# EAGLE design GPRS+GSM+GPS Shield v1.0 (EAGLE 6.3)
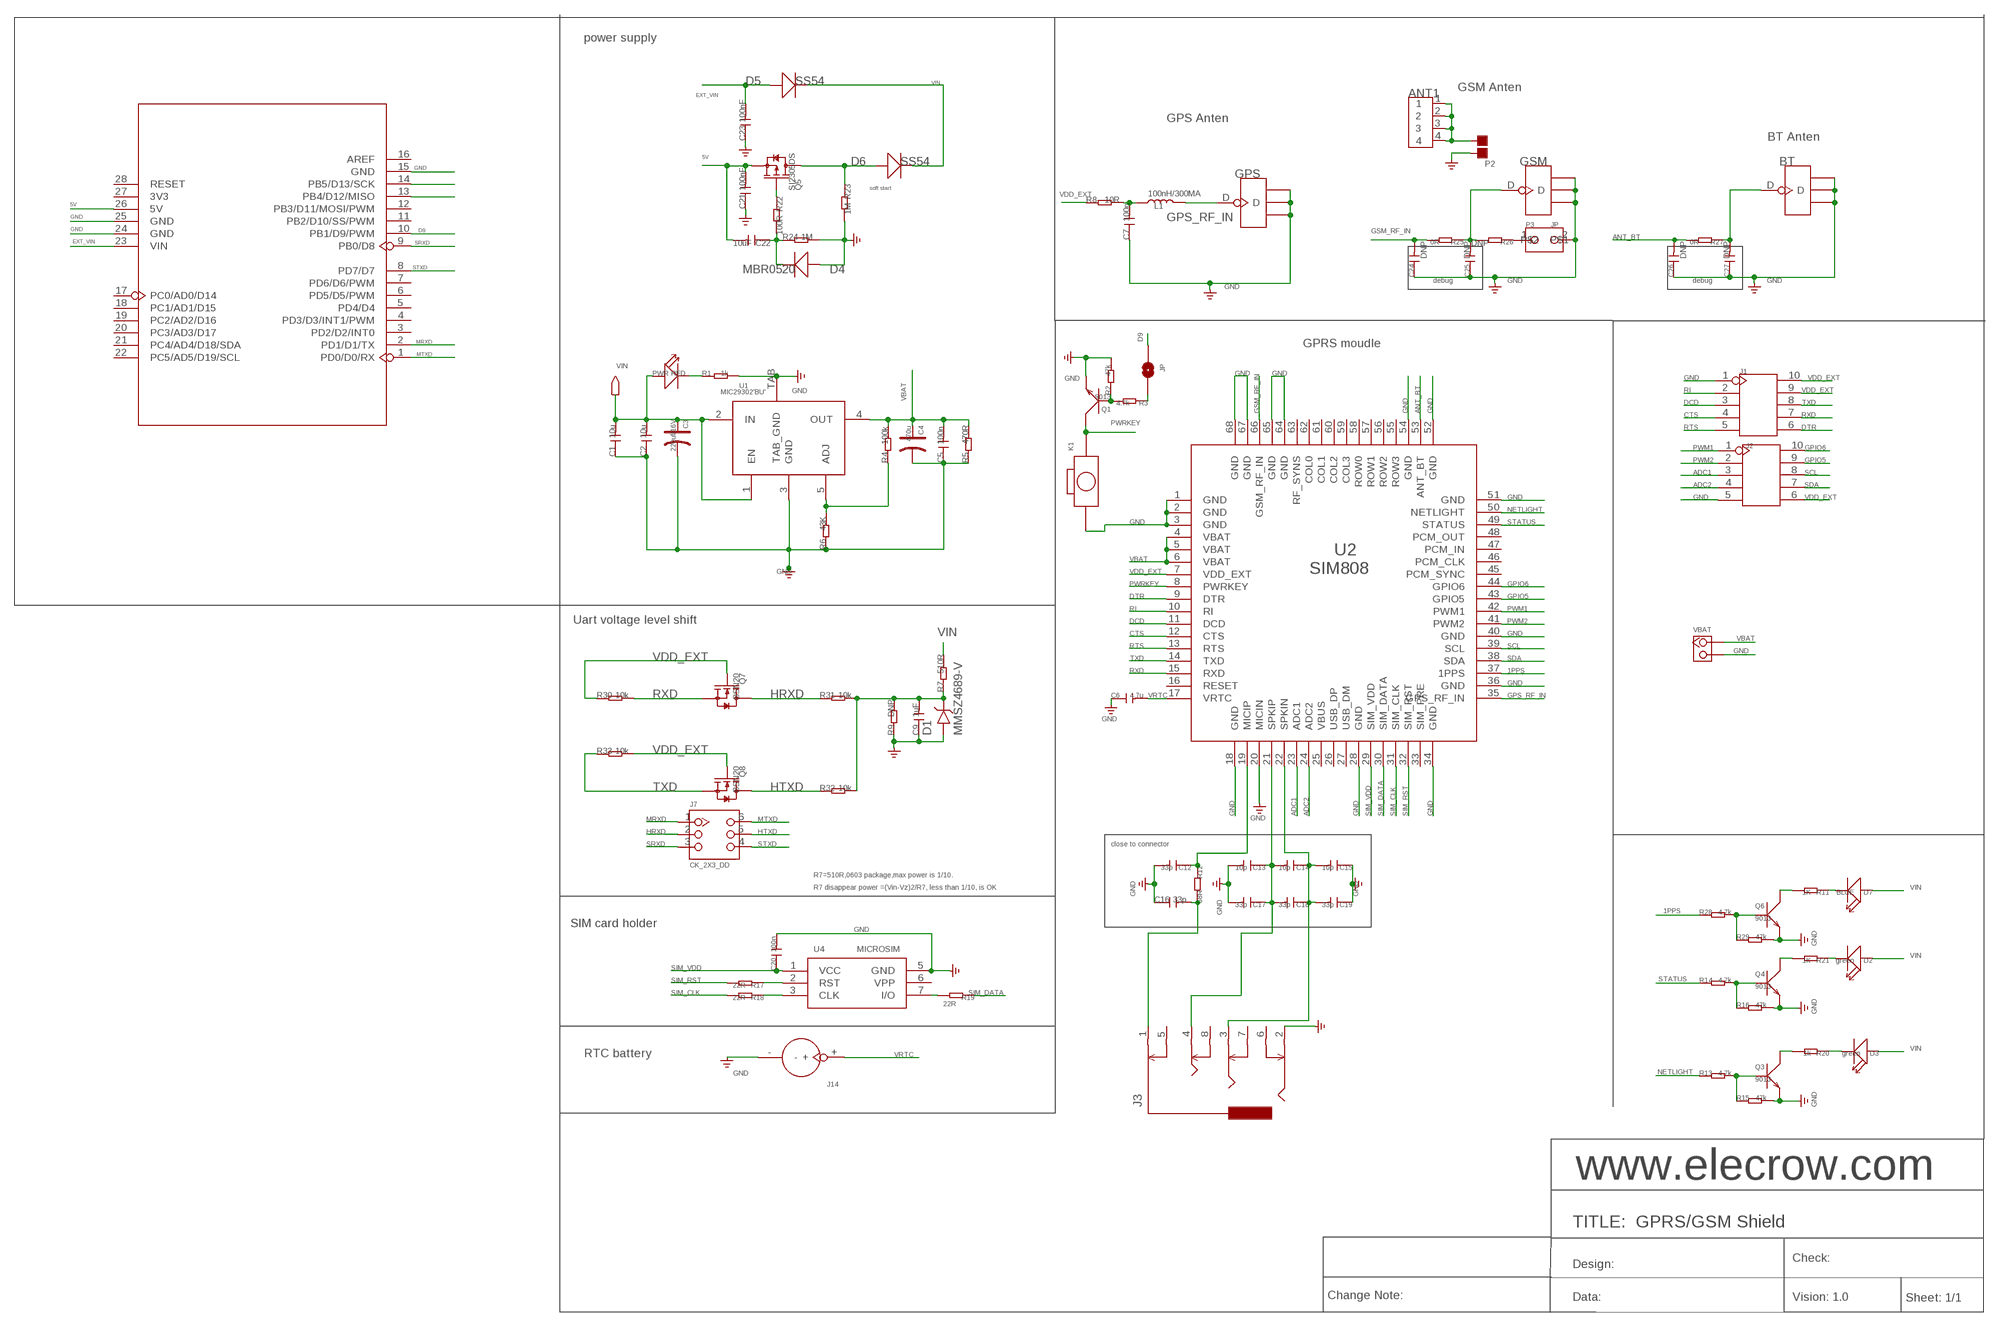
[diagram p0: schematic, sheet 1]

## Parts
ANT1  ANTENNA-SMA-IPX  [SMA-TO-IPX]
BT  ANTENNA-U-FL  [4P-U-FL]
C1  10u  C-0603  [C0603]
C2  10u  C-0603  [C0603]
C3  220uf/16V  006-CAP_AVX_D  [AVX_D]
C4  470u  006-CAP_AVX_D  [AVX_D]
C5  100n  C-0603  [C0603]
C6  4.7u  C-0805  [C0805]
C7  100n  C-0603  [C0603]
C9  1uF  C-0603  [C0603]
C12  33p  C-0603  [C0603]
C13  10p  C-0402  [C0402]
C14  10p  C-0402  [C0402]
C15  10p  C-0402  [C0402]
C16  33p  C-0603  [C0603]
C17  33p  C-0402  [C0402]
C18  33p  C-0402  [C0402]
C19  33p  C-0402  [C0402]
C20  100n  C-0603  [C0603]
C21  100nF  C-0603  [C0603]
C22  10uF  C-0805  [C0805]
C23  100nF  C-0603  [C0603]
C24  DNP  C-0402  [C0402]
C25  DNP  C-0402  [C0402]
C26  DNP  C-0402  [C0402]
C27  DNP  C-0402  [C0402]
D1  MMSZ4689-V  D-VOL'MMSZ4681'  [SOD123-2.7X1.6]
D2  green  LED'0603'  [LED-0603]
D3  green  LED'0603'  [LED-0603]
D4  MBR0520  D'MBR0520LT1'  [SOD123-2.7X1.6]
D5  SS54  D'MBRS240LT3'  [SMB]
D6  SS54  D'MBRS240LT3'  [SMB]
D7  BLUE  LED'0603'  [LED-0603]
GPS  ANTENNA-U-FL  [4P-U-FL]
GSM  ANTENNA-U-FL  [4P-U-FL]
J1  HEADER-2X5P-2.54  [2X5P-2.54]
J2  HEADER-2X5P-2.54  [2X5P-2.54]
J3  AUDIO-8P'PJ-3536-L6S'  [8P-3.5-SMD]
J7  CK_2X3_DD  [CK_2X3]
J14  HOLDER-BATTERY-2P-CR1220  [CR1220]
JP  0R/0805  PAD-SOLDERJUMPERNC  [2P-SMD-3.3X2]
K1  BOTTON_1_DP  [BTN_5.0_RST]
L1  100nH/300MA  L'0603'  [L0603]
P2  PAD-JUMPER-2P  [2P-SMD-1.78X1.27]
P3  JP  [JP]
PWR  RED  007-LED0603  [D0603]
Q1  9013  TRANSISTOR-NPN-SOT23  [SOT23]
Q3  9013  TRANSISTOR-NPN-SOT23  [SOT23]
Q4  9013  TRANSISTOR-NPN-SOT23  [SOT23]
Q5  SI2305DS  MOSFET-P'SI2323CDS/SI2305DS<BR>'  [SOT23]
Q6  9013  TRANSISTOR-NPN-SOT23  [SOT23]
Q7  BSN20  MOSFET-N'SOT23'  [SOT23]
Q8  BSN20  MOSFET-N'SOT23'  [SOT23]
R1  1k  R-0603  [R0603]
R2  47k  R-0603  [R0603]
R3  4.7k  R-0603  [R0603]
R4  100k  R-0603  [R0603]
R5  470R  R-0603  [R0603]
R6  43K  R-0603  [R0603]
R7  510R  R-0603  [R0603]
R8  10R  R-0603  [R0603]
R9  DNP  R-0603  [R0603]
R11  1K  R-0603  [R0603]
R12  68R  R-0603  [R0603]
R13  4.7k  R-0603  [R0603]
R14  4.7k  R-0603  [R0603]
R15  47k  R-0603  [R0603]
R16  47k  R-0603  [R0603]
R17  22R  R-0603  [R0603]
R18  22R  R-0603  [R0603]
R19  22R  R-0603  [R0603]
R20  1k  R-0603  [R0603]
R21  1K  R-0603  [R0603]
R22  100R  R-0603  [R0603]
R23  1M  R-0603  [R0603]
R24  1M  R-0603  [R0603]
R25  0R  R-0402  [R0402]
R26  DNP  R-0402  [R0402]
R27  0R  R-0402  [R0402]
R28  4.7k  R-0603  [R0603]
R29  47k  R-0603  [R0603]
R30  10k  R-0603  [R0603]
R31  10k  R-0603  [R0603]
R32  10k  R-0603  [R0603]
R33  10k  R-0603  [R0603]
U1  MIC29302'BU'  [TO-263]
U2  SIM808  [SIM808]
U3  UNO-SHILED  [SHILED]
U4  MICROSIM  [MICROSIM]
VBAT  DNP  HEADER_1X2_2.54  [CK_1*2]

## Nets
1PPS: R28.1 U2.37(1PPS)
5V: C21.2 C22.2 Q5.2(S) U3.26(5V)
ADC1: J2.3 U2.23(ADC1)
ADC2: J2.4 U2.24(ADC2)
ANT_BT: C26.2 R27.2 U2.53(ANT_BT)
CTS: J1.4 U2.12(CTS)
D9: JP.1 U3.10(PB1/D9/PWM)
DCD: J1.3 U2.11(DCD)
DTR: J1.6 U2.9(DTR)
EXT_VIN: C23.2 D5.+ U3.23(VIN)
GND: BT.GND1 BT.GND2 BT.GND3 C1.1 C2.1 C3.- C4.- C5.1 C6.1 C7.1 C9.1 C12.2 C13.2 C15.1 C16.1 C17.2 C19.1 C20.2 C21.1 C23.1 C24.1 C25.1 C26.1 C27.1 D1.1 D4.1(+) GPS.GND1 GPS.GND2 GPS.GND3 GSM.GND1 GSM.GND2 GSM.GND3 J1.1 J2.5 J3.2 J14.- K1.P$1 P2.2 P3.2 Q1.2(E) Q3.2(E) Q4.2(E) Q6.2(E) R1.2 R2.2 R5.1 R6.1 R9.1 R15.2 R16.2 R23.2 R24.2 R29.2 U1.3(GND) U1.TAB(TAB_GND) U2.1(GND) U2.2(GND) U2.3(GND) U2.18(GND) U2.20(MICIN) U2.28(GND) U2.34(GND) U2.36(GND) U2.40(GND) U2.51(GND) U2.52(GND) U2.54(GND) U2.64(GND) U2.65(GND) U2.67(GND) U2.68(GND) U3.15(GND) U3.24(GND) U3.25(GND) U4.5(GND) VBAT.2
GPIO5: J2.9 U2.43(GPIO5)
GPIO6: J2.10 U2.44(GPIO6)
GPS_RF_IN: GPS.D L1.2 U2.35(GPS_RF_IN)
GSM_RF_IN: C24.2 R25.2 U2.66(GSM_RF_IN)
HRXD: J7.2 Q7.3(D) R31.1
HTXD: J7.5 Q8.3(D) R32.1
MRXD: J7.1 U3.2(PD1/D1/TX)
MTXD: J7.6 U3.1(PD0/D0/RX)
N$1: R19.2 U4.7(I/O)
N$2: R4.1 R6.2 U1.5(ADJ)
N$3: Q3.3(C) R20.2
N$4: Q6.3(C) R11.2
N$5: R18.1 U4.3(CLK)
N$6: R17.1 U4.2(RST)
N$7: D3.- R20.1
N$8: Q3.1(B) R13.2 R15.1
N$9: C9.2 D1.2 R7.1 R9.2 R31.2 R32.2
N$11: Q5.1(G) R22.1
N$12: ANT1.1 ANT1.2 ANT1.3 ANT1.4 P2.1
N$13: C12.1 R12.1 U2.19(MICIP)
N$14: JP.2 R3.1
N$15: C13.1 C14.2 C17.1 C18.2 J3.4 U2.21(SPKIP)
N$16: Q4.3(C) R21.2
N$17: D2.- R21.1
N$18: Q4.1(B) R14.2 R16.1
N$19: C14.1 C15.2 C18.1 C19.2 J3.3 U2.22(SPKIN)
N$20: D6.+ Q5.3(D) R23.1
N$21: C7.2 L1.1 R8.2
N$22: D7.- R11.1
N$23: U3.14(PB5/D13/SCK)
N$24: Q6.1(B) R28.2 R29.1
N$25: C25.2 GSM.D R25.1 R26.2
N$26: P3.1 R26.1
N$27: U3.13(PB4/D12/MISO)
N$28: BT.D C27.2 R27.1
N$30: C16.2 J3.1 R12.2
N$36: Q1.1(B) R2.1 R3.2
N$39: C22.1 D4.2(-) R22.2 R24.1
N$53: PWR.- R1.1
NETLIGHT: R13.1 U2.50(NETLIGHT)
PWM1: J2.1 U2.42(PWM1)
PWM2: J2.2 U2.41(PWM2)
PWRKEY: K1.P$2 Q1.3(C) U2.8(PWRKEY)
RI: J1.2 U2.10(RI)
RTS: J1.5 U2.13(RTS)
RXD: J1.7 Q7.2(S) R30.2 U2.15(RXD)
SCL: J2.8 U2.39(SCL)
SDA: J2.7 U2.38(SDA)
SIM_CLK: R18.2 U2.31(SIM_CLK)
SIM_DATA: R19.1 U2.30(SIM_DATA)
SIM_RST: R17.2 U2.32(SIM_RST)
SIM_VDD: C20.1 U2.29(SIM_VDD) U4.1(VCC)
SRXD: J7.3 U3.9(PB0/D8)
STATUS: R14.1 U2.49(STATUS)
STXD: J7.4 U3.8(PD7/D7)
TXD: J1.8 Q8.2(S) R33.1 U2.14(TXD)
VBAT: C4.+ C5.2 R4.2 R5.2 U1.4(OUT) U2.4(VBAT) U2.5(VBAT) U2.6(VBAT) VBAT.1
VDD_EXT: J1.9 J1.10 J2.6 Q7.1(G) Q8.1(G) R8.1 R30.1 R33.2 U2.7(VDD_EXT)
VIN: C1.2 C2.2 C3.+ D2.+ D3.+ D5.- D6.- D7.+ PWR.+ R7.2 U1.1(EN) U1.2(IN)
VRTC: C6.2 J14.+ U2.17(VRTC)
Unconnected: J3.5 J3.6 J3.7 J3.8 U2.16(RESET) U2.25(VBUS) U2.26(USB_DP) U2.27(USB_DM) U2.33(SIM_PRE) U2.45(PCM_SYNC) U2.46(PCM_CLK) U2.47(PCM_IN) U2.48(PCM_OUT) U3.3(PD2/D2/INT0) U3.4(PD3/D3/INT1/PWM) U3.5(PD4/D4) U3.6(PD5/D5/PWM) U3.7(PD6/D6/PWM) U3.11(PB2/D10/SS/PWM) U3.12(PB3/D11/MOSI/PWM) U3.16(AREF) U3.17(PC0/AD0/D14) U3.18(PC1/AD1/D15) U3.19(PC2/AD2/D16) U3.20(PC3/AD3/D17) U3.21(PC4/AD4/D18/SDA) U3.22(PC5/AD5/D19/SCL) U3.27(3V3) U3.28(RESET) U4.6(VPP)

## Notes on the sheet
- power supply
- GSM Anten
- GPS Anten
- BT Anten
- soft start
- debug | debug
- GPRS moudle
- Uart voltage level shift
- close to connector
- R7=510R,0603 package,max power is 1/10.
- R7 disappear power =(Vin-Vz)2/R7, less than 1/10, is OK
- SIM card holder
- RTC battery
- www.elecrow.com
- TITLE:  GPRS/GSM Shield
- Check:
- Design:
- Change Note: | Data: | Vision: 1.0 | Sheet: 1/1

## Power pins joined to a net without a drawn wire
COL0: U2.62(COL0)
COL1: U2.61(COL1)
COL2: U2.60(COL2)
COL3: U2.59(COL3)
RF_SYNS: U2.63(RF_SYNS)
ROW0: U2.58(ROW0)
ROW1: U2.57(ROW1)
ROW2: U2.56(ROW2)
ROW3: U2.55(ROW3)

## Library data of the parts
ANT1 = Connector:ANTENNA-SMA-IPX
BT GPS GSM = Connector:ANTENNA-U-FL
C1 C2 C5-C7 C9 C12-C27 = Discrete:C*: Ceramic Capacitors
C3 C4 = Discrete:006-CAP*: Electrolytic Capacitors,Tantalum Capacitors and Super Capacitors
D1 = template:D-VOL
D2 D3 D7 = Discrete:LED*
D4-D6 = Discrete:D*
J1 J2 = Connector:HEADER-2X5P
J3 = template:AUDIO-8P
J7 = CONNECTER:CK_2X3
J14 = Connector:HOLDER-BATTERY-2P
JP = Discrete:PAD-SOLDERJUMPER: Solder Jumper
K1 = CPT_SMD:BOTTON_1
L1 = Discrete:L*
P2 = Discrete:PAD-JUMPER-2P; PARTNO: DNP
P3 = mySeeed:JP
PWR = Discrete:007-LED*
Q1 Q3 Q4 Q6 = Discrete:TRANSISTOR-NPN*: NPN audion
Q5 = Discrete:MOSFET-P
Q7 Q8 = Discrete:MOSFET-N: IRLL014: http://www.vishay.com/docs/91319/sihll014.pdf
R1-R9 R11-R33 = Discrete:R*
U1 = ICs_v54:MIC29302
U2 = moudle:SIM808
U3 = ljb:UNO-SHILED
U4 = Connector:MICROSIM
VBAT = CONNECTER:HEADER_1X2

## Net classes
0 default: width 0.152 mm, drill 0.152 mm, clearance 0.152 mm

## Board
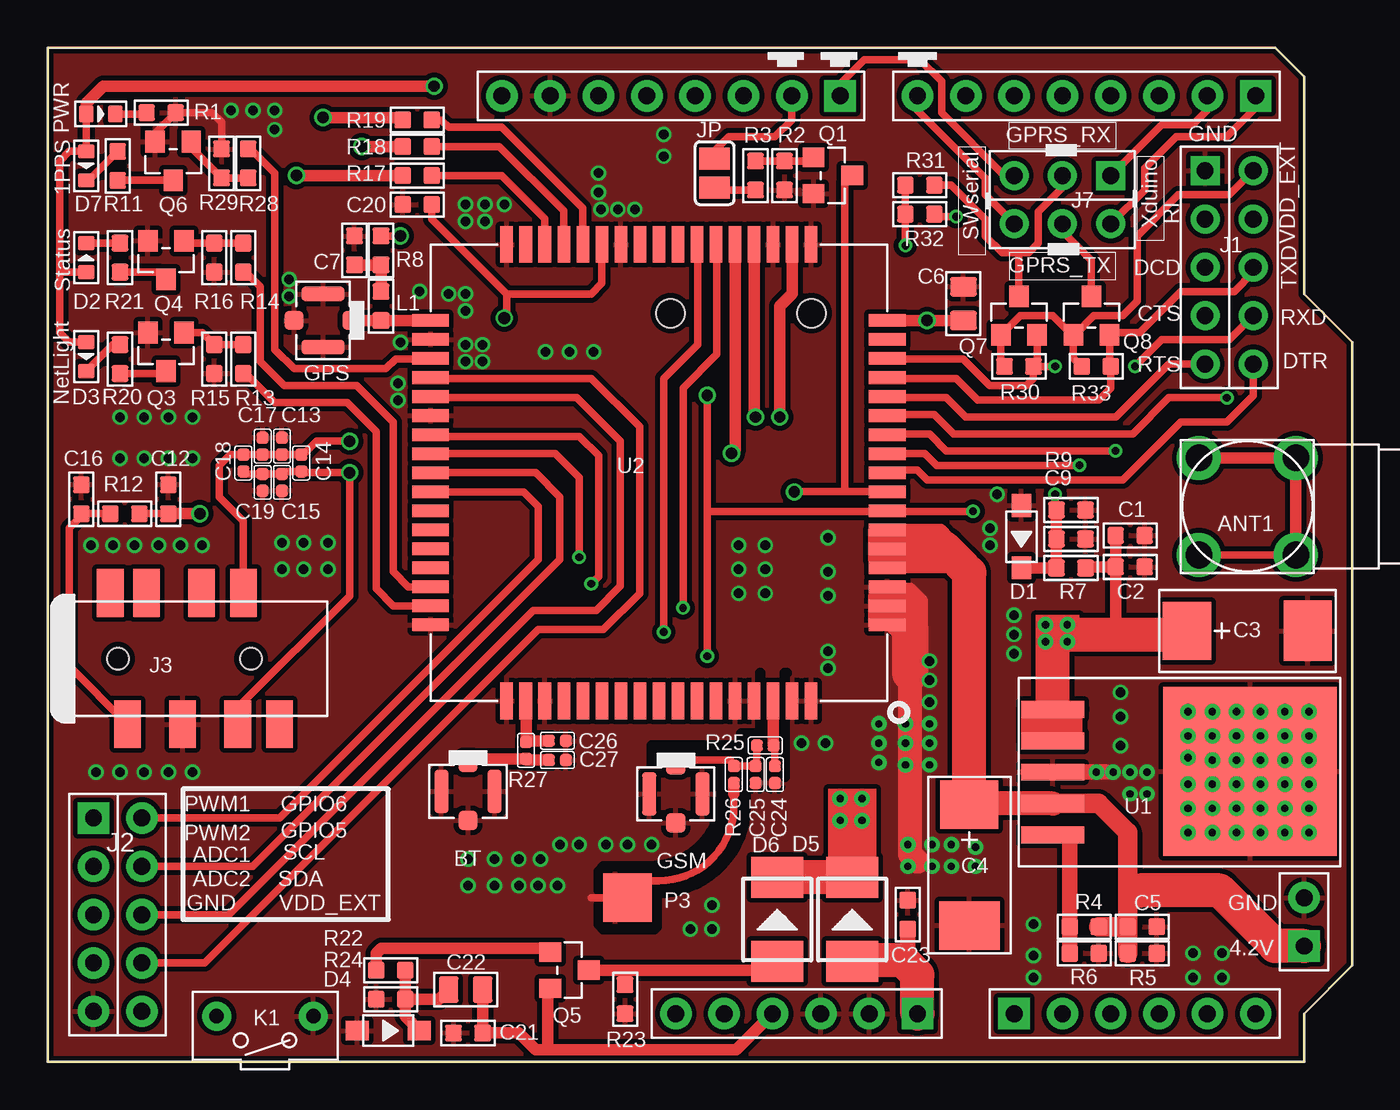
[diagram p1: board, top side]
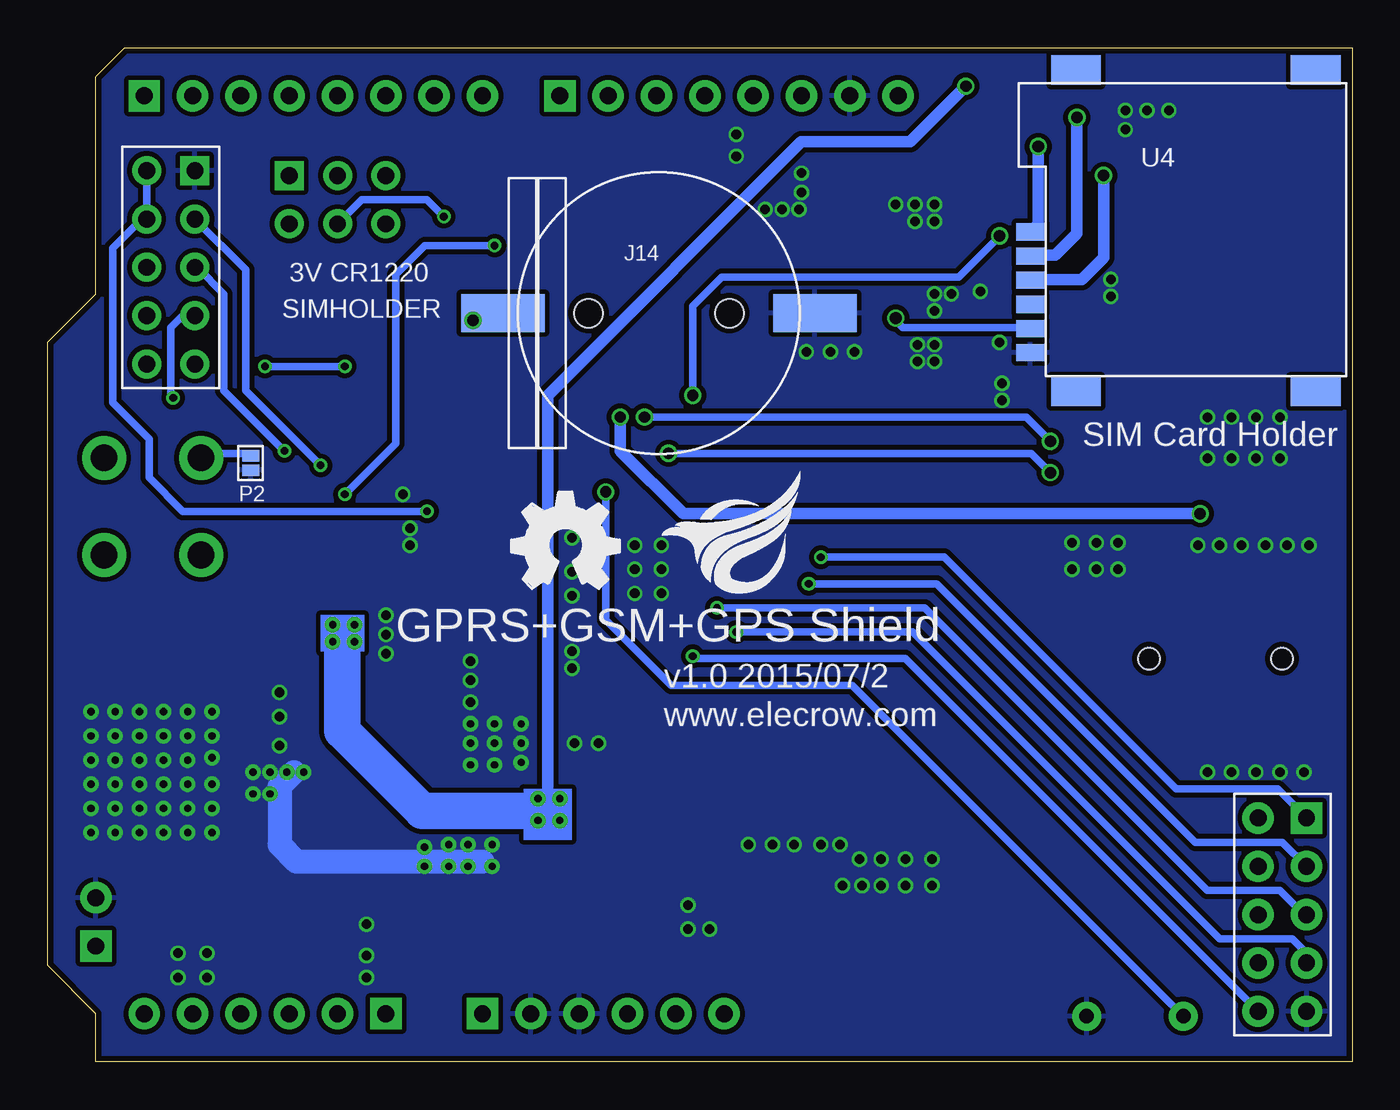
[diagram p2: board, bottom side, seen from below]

Size 68.58 x 53.34 mm. Coordinates in mm from the lower left corner, seen from the top.
Outline: 0,0 66.04,0 66.04,2.54 68.58,5.08 68.58,37.85 66.04,40.39 66.04,51.82 64.52,53.34 0,53.34 0,0
Copper layers (1*16): Top 0.035mm / dielectric 1.5mm / Bottom 0.035mm
Design rules "default *": minimum track width 6mil, minimum drill 12mil, track to track 10mil, track to pad 10mil, pad to pad 10mil, via to via 6mil, smd to smd 0mil, copper to edge 12mil, drill to drill 12mil, minimum pad ring 10mil, minimum via ring 6mil, stop-mask expansion 2mil, vias tented up to drill 100mil, thermal gap 10mil
tRestrict: area 35.6,41.9 to 35.7,43.3; 19 lines

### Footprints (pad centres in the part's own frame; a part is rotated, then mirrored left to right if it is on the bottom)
SMA-TO-IPX = drill 1.4 pad 2.3: 1 -2.55,2.55; 2 2.55,2.55; 3 2.55,-2.55; 4 -2.55,-2.55
4P-U-FL = smd 1.016 x 1.016: D -1.524,0; GND3 1.524,0 | smd 2.286 x 0.762: GND1 0,1.397; GND2 0,-1.397
C0603 = smd 0.889 x 0.889: 1 -0.762,0; 2 0.762,0
AVX_D = smd 2.54 x 3.048: + -3.175,0 | smd 2.54 x 3.175: - 3.175,0
C0805 = smd 1.016 x 1.397: 1 -0.889,0; 2 0.889,0
C0402 = smd 0.635 x 0.635: 1 -0.445,0; 2 0.445,0
SOD123-2.7X1.6 = smd 1.2 x 1.02: 1 -1.635,0; 2 1.635,0
D0603 = smd 0.762 x 0.889: + -0.762,0; - 0.762,0
SMB = smd 2.159 x 2.743: + -2.21,0; - 2.21,0
LED-0603 = smd 0.762 x 0.889: + -0.762,0; - 0.762,0
U-FL = smd 1.016 x 1.016: D -1.524,0; GND3 1.524,0 | smd 2.286 x 0.762: GND1 0,1.397; GND2 0,-1.397
2X5P-2.54-LEADED = drill 0.889 pad 1.524 square: 1 -1.27,5.08 | drill 0.889 pad 1.524: 2 -1.27,2.54; 3 -1.27,0; 4 -1.27,-2.54; 5 -1.27,-5.08; 6 1.27,-5.08; 7 1.27,-2.54; 8 1.27,0; 9 1.27,2.54; 10 1.27,5.08
2X5P-2.54 = drill 0.889 pad 1.651 square: 1 -1.27,5.08 | drill 0.889 pad 1.651: 2 -1.27,2.54; 3 -1.27,0; 4 -1.27,-2.54; 5 -1.27,-5.08; 6 1.27,-5.08; 7 1.27,-2.54; 8 1.27,0; 9 1.27,2.54; 10 1.27,5.08
8P-3.5-SMD = smd 1.4 x 2.5: 1 2.8,-3.45; 2 5.7,-3.45; 3 8.6,-3.45; 4 8.9,3.45; 5 1.9,3.45; 6 3.8,3.45; 7 6.7,3.45; 8 10.8,-3.45 | hole 1.149: 2.3,0; 9.3,0
CK_2X3 = drill 0.889 pad 1.524 square: 1 -1.27,2.54 | drill 0.889 pad 1.524: 2 -1.27,0; 3 -1.27,-2.54; 4 1.27,-2.54; 5 1.27,0; 6 1.27,2.54
CR1220 = smd 2 x 4.4: + 0,-8.2; - 0,8.2 | hole 1.5: 0,3.7; 0,-3.7
2P-SMD-3.3X2 = smd 1.168 x 1.6: 1 -0.762,0; 2 0.762,0
BTN_5.0_RST = drill 0.762 pad 1.524: P$1 0,2.54; P$2 0,-2.54
L0603 = smd 0.889 x 0.889: 1 -0.762,0; 2 0.762,0
2P-SMD-1.78X1.27 = smd 0.889 x 0.61: 1 0,0.381; 2 0,-0.381
JP = smd 1.27 x 2.54: 1 -0.635,0; 2 0.635,0
SOT23 = smd 1.016 x 1.143: 1 -0.95,-1.016; 2 0.95,-1.016; 3 0,1.016
R0603 = smd 0.889 x 0.889: 1 -0.762,0; 2 0.762,0
R0402 = smd 0.635 x 0.635: 1 -0.445,0; 2 0.445,0
TO-263 = smd 3.302 x 0.889: 1 3.302,-3.302; 2 3.302,-1.651; 3 3.302,0; 4 3.302,1.651; 5 3.302,3.302 | smd 9.12 x 8.89: TAB -7.071,-0.03
SIM808 = smd 1.93 x 0.66: 1 -10.349,7.238; 2 -10.349,6.238; 3 -10.349,5.238; 4 -10.349,4.238; 5 -10.349,3.238; 6 -10.349,2.238; 7 -10.349,1.238; 8 -10.349,0.238; 9 -10.349,-0.762; 10 -10.349,-1.762; 11 -10.349,-2.762; 12 -10.349,-3.762; 13 -10.349,-4.762; 14 -10.349,-5.762; 15 -10.349,-6.762; 16 -10.349,-7.762; 17 -10.349,-8.762; 35 13.651,-8.762; 36 13.651,-7.762; 37 13.651,-6.762; 38 13.651,-5.762; 39 13.651,-4.762; 40 13.651,-3.762; 41 13.651,-2.762; 42 13.651,-1.762; 43 13.651,-0.762; 44 13.651,0.238; 45 13.651,1.238; 46 13.651,2.238; 47 13.651,3.238; 48 13.651,4.238; 49 13.651,5.238; 50 13.651,6.238; 51 13.651,7.238 | smd 0.66 x 1.93: 18 -6.349,-12.762; 19 -5.349,-12.762; 20 -4.349,-12.762; 21 -3.349,-12.762; 22 -2.349,-12.762; 23 -1.349,-12.762; 24 -0.349,-12.762; 25 0.651,-12.762; 26 1.651,-12.762; 27 2.651,-12.762; 28 3.651,-12.762; 29 4.651,-12.762; 30 5.651,-12.762; 31 6.651,-12.762; 32 7.651,-12.762; 33 8.651,-12.762; 34 9.651,-12.762; 52 9.651,11.238; 53 8.651,11.238; 54 7.651,11.238; 55 6.651,11.238; 56 5.651,11.238; 57 4.651,11.238; 58 3.651,11.238; 59 2.651,11.238; 60 1.651,11.238; 61 0.651,11.238; 62 -0.349,11.238; 63 -1.349,11.238; 64 -2.349,11.238; 65 -3.349,11.238; 66 -4.349,11.238; 67 -5.349,11.238; 68 -6.349,11.238
SHILED = drill 0.889 pad 1.651 square: 1 63.5,50.8; 9 41.656,50.8; 17 50.8,2.54; 23 45.72,2.54 | drill 0.889 pad 1.651: 2 60.96,50.8; 3 58.42,50.8; 4 55.88,50.8; 5 53.34,50.8; 6 50.8,50.8; 7 48.26,50.8; 8 45.72,50.8; 10 39.116,50.8; 11 36.576,50.8; 12 34.036,50.8; 13 31.496,50.8; 14 28.956,50.8; 15 26.416,50.8; 16 23.876,50.8; 18 53.34,2.54; 19 55.88,2.54; 20 58.42,2.54; 21 60.96,2.54; 22 63.5,2.54; 24 43.18,2.54; 25 40.64,2.54; 26 38.1,2.54; 27 35.56,2.54; 28 33.02,2.54
MICROSIM = smd 1.5 x 0.9: 1 -0.8,2.5; 2 -0.8,5.04; 3 -0.8,7.58; 5 -0.8,1.23; 6 -0.8,3.77; 7 -0.8,6.31 | smd 2.61 x 1.56: P$1 1.6,-0.8; P$2 14.2,-0.8; P$3 14.2,16.1; P$4 1.6,16.1
CK_1*2 = drill 0.889 pad 1.651 square: 1 0,1.27 | drill 0.889 pad 1.651: 2 0,-1.27

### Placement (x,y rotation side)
ANT1  63.06,29.21 90 top
BT  22.1,14.22 270 top
C1  56.9,27.69 180 top
C2  56.9,26.04 180 top
C3  63.06,22.67 0 top
C4  48.45,10.35 270 top
C5  57.53,7.11 180 top
C6  48.13,39.88 270 top
C7  16.13,42.67 270 top
C9  53.78,27.5 180 top
C12  6.35,29.59 90 top
C13  12.32,32.38 90 top
C14  13.34,31.5 90 top
C15  12.32,30.48 90 top
C16  1.78,29.59 270 top
C17  11.3,32.38 90 top
C18  10.29,31.5 90 top
C19  11.3,30.48 90 top
C20  19.43,45.09 180 top
C21  22.1,1.52 0 top
C22  21.97,3.81 0 top
C23  45.21,7.75 270 top
C24  38.23,15.11 90 top
C25  37.21,15.11 90 top
C26  26.8,16.89 180 top
C27  26.8,15.88 180 top
D1  51.18,27.62 270 top
D2  green  [D0603]  2.03,42.29 90 top
D3  green  [D0603]  2.03,37.08 270 top
D4  17.91,1.65 0 top
D5  42.29,7.49 90 top
D6  38.35,7.49 90 top
D7  2.03,47.12 270 top
GPS  [U-FL]  14.48,38.99 180 top
GSM  33.02,14.1 270 top
J1  [2X5P-2.54-LEADED]  62.1,41.78 0 top
J2  3.68,7.75 0 top
J3  1.4,21.21 0 top
J7  53.34,45.34 270 top
J14  36.45,39.37 270 bottom
JP  35.05,46.74 270 top
K1  11.43,2.41 270 top
L1  17.53,39.75 270 top
LOGO2  LOGO-OSHW-FILLX0200-NT  [OSHW_FILLX200_NOTEXT]  44.2,24.89 0 bottom
P2  57.91,31.5 0 bottom
P3  30.48,8.64 180 top
PWR  2.79,49.85 0 top
Q1  41.27,46.61 270 top
Q3  6.22,37.34 180 top
Q4  6.22,42.16 180 top
Q5  27.43,4.83 270 top
Q6  6.6,47.37 180 top
Q7  51.05,39.24 0 top
Q8  54.86,39.24 0 top
R1  5.97,49.91 0 top
R2  38.73,46.61 270 top
R3  37.21,46.61 90 top
R4  54.48,7.11 0 top
R5  57.53,5.71 180 top
R6  54.48,5.71 180 top
R7  53.78,25.97 0 top
R8  17.53,42.67 270 top
R9  53.78,29.02 180 top
R11  3.68,47.12 270 top
R12  4.06,28.83 180 top
R13  10.29,36.96 90 top
R14  10.29,42.29 90 top
R15  8.76,36.96 270 top
R16  8.76,42.29 270 top
R17  19.43,46.61 0 top
R18  19.43,48.13 0 top
R19  19.43,49.53 180 top
R20  3.81,36.96 270 top
R21  3.81,42.29 270 top
R22  18.03,4.83 0 top
R23  30.35,3.3 270 top
R24  18.03,3.3 180 top
R25  37.72,16.64 0 top
R26  36.07,15.11 90 top
R27  25.15,16.38 90 top
R28  10.54,47.24 270 top
R29  9.14,47.24 90 top
R30  51.05,36.58 0 top
R31  45.85,46.1 180 top
R32  45.85,44.58 180 top
R33  55.12,36.58 180 top
U1  56.13,15.24 180 top
U2  33.78,30.23 180 top
U3  0,0 0 top
U4  16.13,36.07 0 bottom
U$4  [ELECROW_NRW_6]  36.32,24.64 0 bottom
VBAT  66.04,7.37 180 top

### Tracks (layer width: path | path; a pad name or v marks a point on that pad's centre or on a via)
1PPS
  Top 0.406: U2.37 20.1,36.96 18.29,36.96 17.78,36.45 12.95,36.45 11.94,37.47 11.94,46.74 10.67,48.01 R28.1
5V
  Top 0.61: C22.2 C21.2 24.77,1.52 25.65,0.64 26.29,0.64 | U3.26 36.2,0.64 26.29,0.64 | Q5.2 26.29,3.75 26.29,0.64
ADC1  (via drill 0.41)
  Top 0.406: U2.23 35.18,42.94 35.18,37.21 33.4,35.43 v33.4,23.88
  Bottom 0.406: J2.3 2.54,7.75 3.81,9.02 7.62,9.02 22.48,23.88 v33.4,23.88
ADC2  (via drill 0.41)
  Top 0.406: U2.24 34.16,42.96 34.16,37.72 32.38,35.94 v32.38,22.61
  Bottom 0.406: 32.26,22.73 v32.38,22.61 23.11,22.61 6.99,6.48 3.17,6.48 2.41,5.71 J2.4
ANT_BT
  Top 0.61: U2.53 25.15,18.99 R27.2 25.15,16.89 C26.2
CTS  (via drill 0.41)
  Top 0.406: U2.12 44.18,34.04 46.61,34.04 47.62,33.02 57.02,33.02 58.93,34.92 v61.98,34.92
  Bottom 0.406: v61.98,34.92 62.1,35.05 62.1,38.61 61.47,39.24 J1.4
D9
  Top 0.406: JP.1 35.05,47.88 35.81,48.64 38.23,48.64 39.12,49.53 U3.10
DCD  (via drill 0.41)
  Top 0.406: U2.11 44.16,33.02 46.35,33.02 47.24,32.13 v56.13,32.13
  Bottom 0.406: v56.13,32.13 59.31,35.31 59.31,40.39 60.71,41.78 J1.3
DTR
  Top 0.406: U2.9 44.26,31.11 45.72,31.11 46.23,30.61 56.52,30.61 59.56,33.66 61.98,33.66 63.37,35.05 J1.6
EXT_VIN
  Top 0.813: C23.2 45.21,5.59 44.96,5.33
  Top 1.778: U3.23 45.72,4.57 44.96,5.33 42.34,5.33 D5.+
GND  (via drill 0.38 pad 0.81, 0.5)
  Top 0.406: Q6.2 5.65,48.83 R1.2 8.64,49.91 9.14,49.4 R29.2 | P3.2 28.57,8.64
  Top 0.61: U2.1 U2.2 U2.3 44.23,24.89 45.34,24.89 45.97,24.26 45.97,20.45 45.59,20.83 45.59,24.26 45.21,24.64 44.83,24.64 44.7,24.51 43.43,24.51 43.43,22.99 44.45,22.99 45.47,21.97 45.47,20.32 45.34,20.45
  Top 0.813: U1.3 55.63,15.24 | 45.47,20.32 45.47,20.19
  Top 1.27: 45.72,10.54 45.34,10.92 45.34,20.45
  Top 1.93: U2.2 45.34,22.78 45.34,20.45
  Bottom 1.27: 55.63,15.24 56.39,14.48 56.39,11.43 55.5,10.54 45.72,10.54
  other vias: 59.94,18.41 59.94,17.14 59.94,13.34 59.94,12.06 61.21,12.06 62.48,12.06 63.75,12.06 65.02,12.06 66.29,12.06 66.29,13.34 66.29,14.61 66.29,15.88 66.29,17.14 66.29,18.41 63.75,13.34 63.75,14.61 63.75,15.88 63.75,17.14 63.75,18.41 65.02,13.34 65.02,14.61 65.02,15.88 65.02,17.14 65.02,18.41 62.48,13.34 62.48,14.61 62.48,15.88 62.48,17.14 62.48,18.41 61.21,13.34 61.21,14.61 61.21,15.88 61.21,17.14 61.21,18.41 59.94,16 59.94,14.61 22.86,37.72 18.41,35.69 56.39,16.64 56.39,18.16 56.39,19.43 39.62,16.76 40.89,16.76 22.1,10.67 23.5,10.67 24.77,10.67 22.1,9.27 23.5,9.27 24.77,9.27 60.2,5.71 61.72,5.71 60.2,4.45 61.72,4.45 51.82,7.24 51.82,5.59 51.82,4.45 3.81,31.75 22.99,45.09 22.99,44.2 21.97,44.2 21.97,45.09 24,45.09 41.02,27.56 41.02,25.78 41.02,24.51 41.02,20.7 41.02,21.59 37.72,27.18 37.72,25.91 37.72,24.64 36.32,24.64 36.32,25.91 36.32,27.18 14.73,25.91 13.46,25.91 2.54,15.24 34.92,8.26 34.92,6.99 33.78,6.99 32.38,48.77 32.38,47.62 29.97,44.83 29.08,44.83 45.09,16.76 45.09,15.62 45.09,17.78 46.35,17.78 46.35,16.76 46.35,15.62 43.69,17.78 43.69,16.76 43.69,15.75 46.48,11.43 45.21,11.43 45.21,10.29 46.48,10.29 47.5,10.29 47.5,11.43 48.77,10.29 48.77,11.3 56.9,15.24 56.9,14.1 55.12,15.24 56.01,15.24 57.78,15.24 57.78,14.1 46.35,18.92 46.35,20.07 46.35,21.08 3.81,15.24 5.08,15.24 6.35,15.24 7.62,15.24 12.32,25.91 12.32,27.3 13.46,27.3 14.73,27.3 5.08,31.75 6.35,31.75 7.62,31.75 5.08,33.91 6.35,33.91 7.62,33.91 3.81,33.91 18.41,34.8 21.97,37.72 21.97,36.83 18.54,37.85 12.7,41.15 12.7,40.26 21.97,39.5 21.97,40.39 21.08,40.39 19.56,40.51 22.86,36.83 30.86,44.83 28.96,45.72 28.96,46.74 31.75,11.43 30.48,11.43 29.34,11.43 27.94,11.43 26.92,11.43 25.91,10.67 25.78,9.27 26.8,9.27 8.13,27.18 6.99,27.18 5.84,27.18 4.57,27.18 3.43,27.18 2.29,27.18 28.7,37.34 27.43,37.34 26.16,37.34 9.65,50.04 10.79,50.04 11.94,50.04 11.94,49.02 49.91,29.84 49.53,28.07 49.53,27.18 50.8,23.5 50.8,22.48 50.8,21.46
  pour Bottom (isolate 0.254): -1.27,-1.27 71.12,-1.27 71.12,54.61 -1.27,54.61
  pour Top (isolate 0.254): -1.27,-1.27 71.12,-1.27 71.12,54.61 -1.27,54.61
GPIO5
  Top 0.406: U2.43 25.65,30.99 26.92,29.72 26.92,26.42 10.79,10.29 J2.9
GPIO6
  Top 0.406: U2.44 20.15,29.97 25.02,29.97 25.78,29.21 25.78,26.42 12.19,12.83 J2.10
GPS_RF_IN
  Top 0.61: U2.35 L1.2 GPS.D
GSM_RF_IN
  Top 0.406: C24.2 38.23,16.57 R25.2 38.13,16.67
  Top 0.61: 38.13,16.67 U2.66
HRXD
  Top 0.406: J7.2 53.34,45.97 52.07,44.7 52.07,43.05 51.56,42.55 51.05,42.55 | R31.1 46.74,45.97 46.86,46.1 47.5,46.1 49.28,44.32 49.28,43.43 50.16,42.55 51.05,42.55 | Q7.3 51.05,42.55
HTXD  (via drill 0.41)
  Top 0.406: J7.5 53.34,43.69 54.86,42.16 Q8.3 | R32.1 46.74,44.45 v47.75,44.45
  Bottom 0.406: v47.75,44.45 48.64,45.34 52.07,45.34 J7.5
MRXD
  Top 0.406: J7.1 58.55,49.28 60.2,49.28 60.96,50.04 U3.2
MTXD
  Top 0.406: J7.6 57.66,45.85 57.66,46.99 59.31,48.64 61.98,48.64 63.5,50.16 U3.1
N$1  (via drill 0.61)
  Top 0.61: R19.2 18.54,49.66 v14.48,49.66
  Bottom 0.61: v14.48,49.66 14.48,43.56 15.62,42.42 16.89,42.42 U4.7
N$2
  Top 0.813: R6.2 R4.1 53.72,11.94 U1.5
N$3
  Top 0.406: Q3.3 6.1,36.2 R20.2
N$4
  Top 0.406: R11.2 Q6.3
N$5  (via drill 0.61)
  Top 0.61: R18.1 v16.51,48.13
  Bottom 0.61: U4.3 16.51,44.07 v16.51,48.13
N$6  (via drill 0.61)
  Top 0.61: R17.1 v13.08,46.61
  Bottom 0.61: v13.08,46.61 13.08,42.29 14.22,41.15 16.89,41.15 U4.2
N$7
  Top 0.406: D3.- 3.43,37.72 R20.1
N$8
  Top 0.406: R13.2 R15.1 8.13,38.35 Q3.1
N$9  (via drill 0.41)
  Top 0.254: 53.01,25.99 R7.1
  Top 0.406: R31.2 R32.2 v45.09,42.93 | R9.2 52.96,29.08 v52.96,29.84
  Top 0.61: D1.2 53.01,25.99 | R7.1 C9.2 R9.2
  Bottom 0.406: v52.96,29.84 50.29,32.51 50.29,41.4 48.77,42.93 v45.09,42.93
N$11
  Top 0.406: 26.22,5.97 Q5.1
  Top 0.61: R22.1 17.27,5.71 17.53,5.97 26.22,5.97
N$12
  Top 0.406: ANT1.1 ANT1.4
  Top 0.61: ANT1.4 ANT1.3 ANT1.2
  Bottom 0.406: P2.1 58.04,32 59.94,32 60.19,31.76 ANT1.2
N$13  (via drill 0.6)
  Top 0.406: C12.1 R12.1
  Top 0.61: v38.48,33.91 38.48,39.75 39.13,40.4 U2.19 | C12.1 v8,28.83
  Bottom 0.61: v8,28.83 35.18,28.83 38.48,32.13 v38.48,33.91
N$14
  Top 0.406: R3.1 35.18,45.85 JP.2
N$15  (via drill 0.6)
  Top 0.406: v15.88,32.64 14.16,32.64 13.4,31.88 C14.2 C13.1 C17.1 C18.2 9.59,31.94 9.02,31.37 9.02,29.72 10.29,28.45 10.29,24.67 J3.4
  Top 0.61: v37.21,33.91 37.13,33.99 U2.21
  Bottom 0.406: v37.21,33.91 17.14,33.91 v15.88,32.64
N$16
  Top 0.406: Q4.3 5.84,41.53 R21.2
N$17
  Top 0.406: D2.- R21.1
N$18
  Top 0.406: Q4.1 7.3,43.05 R16.1 R14.2
N$19  (via drill 0.6)
  Top 0.305: C18.1 10.41,30.92 | C15.2 12.45,31.05
  Top 0.406: J3.3 10.16,17.92 10.16,18.8 15.88,24.51 v15.88,30.99 13.4,30.99 C14.1 12.45,31.05 | 10.41,30.92 C19.2 C15.2
  Top 0.61: v35.94,32 36.13,32.19 U2.22
  Bottom 0.406: v15.88,30.99 16.89,32 v35.94,32
N$20
  Top 0.406: 37.9,4.83 D6.+
  Top 0.61: Q5.3 30.35,4.83 | 30.35,4.83 37.9,4.83 | R23.1 30.35,4.83
N$21
  Top 0.61: L1.1 R8.2 C7.2
N$22
  Top 0.406: D7.- 2.16,46.35 R11.1
N$24
  Top 0.406: Q6.1 7.55,48.07 R29.1 R28.2
N$25
  Top 0.406: GSM.D 33.27,15.88 35.88,15.88 R26.2 C25.2 37.27,15.62 R25.1
N$26
  Top 0.406: 36.07,14.1 36.07,13.46 arc-90 32.13,9.53 31.5,9.53 arc90 31.37,9.4 31.37,8.89 arc-90 P3.1
  Top 0.61: R26.1 36.07,14.1
N$28
  Top 0.61: C27.2 25.15,15.88 R27.1 22.1,15.94 BT.D
N$30
  Top 0.406: C16.2 R12.2 3.04,28.57 | J3.1 1.14,20.81 1.14,28.07 1.78,28.7 C16.2 | 1.78,28.57 C16.2
N$36
  Top 0.406: R3.2 R2.1 40.07,47.37 Q1.1
N$39
  Top 0.61: R24.1 R22.2 | R24.1 20.57,3.3 C22.1 | D4.2 18.8,2.4 R24.1
N$53
  Top 0.406: PWR.- 5.21,49.85 R1.1
NETLIGHT
  Top 0.406: U2.50 18.18,23.99 17.27,24.89 17.27,33.15 15.75,34.67 11.94,34.67 10.41,36.2 R13.1
PWM1  (via drill 0.41)
  Top 0.406: U2.42 20.15,32 26.67,32 27.94,30.73 v27.94,26.54
  Bottom 0.406: J2.1 3.94,14.35 9.27,14.35 21.46,26.54 v27.94,26.54
PWM2  (via drill 0.41)
  Top 0.406: U2.41 20.23,32.89 27.94,32.89 28.96,31.88 28.96,25.53 v28.57,25.15
  Bottom 0.406: J2.2 3.68,11.56 8.26,11.56 21.84,25.15 v28.57,25.15
PWRKEY  (via drill 0.6)
  Top 0.406: Q1.3 41.91,46.23 41.91,29.99 | 43.04,29.99 U2.8 | U2.8 44.12,29.97 | v39.24,29.97 39.26,29.99 41.91,29.99 | 41.91,29.99 U2.8
  Bottom 0.406: K1.P$2 26.29,19.81 35.81,19.81 39.24,23.24 v39.24,29.97
RI  (via drill 0.41)
  Top 0.406: U2.10 44.15,32 46.1,32 46.74,31.37 v54.23,31.37
  Bottom 0.406: v54.23,31.37 58.17,35.31 58.17,41.66 J1.2
RTS
  Top 0.406: U2.13 44.19,34.92 47.24,34.92 48.26,33.91 56.13,33.91 58.93,36.7 J1.5
RXD  (via drill 0.41)
  Top 0.406: R30.2 52,36.76 Q7.2 | U2.15 44.16,36.96 48.13,36.96 49.53,35.56 51.44,35.56 51.82,35.94 R30.2 | J1.7 62.1,37.97 58.55,37.97 v57.15,36.58 | v52.96,36.58 R30.2
  Bottom 0.406: v52.96,36.58 v57.15,36.58
SCL
  Top 0.406: U2.39 20.19,34.92 27.81,34.92 30.1,32.64 30.1,25.02 28.83,23.75 25.53,23.75 9.53,7.75 J2.8
SDA
  Top 0.406: U2.38 20.18,35.94 28.57,35.94 31.11,33.4 31.11,24.64 29.21,22.73 25.78,22.73 8.26,5.21 J2.7
SIM_CLK
  Top 0.406: U2.31 27.13,44.75 23.75,48.13 R18.2
SIM_DATA
  Top 0.406: U2.30 28.13,44.89 23.88,49.15 21.08,49.15 20.7,49.53 R19.1
SIM_RST
  Top 0.406: U2.32 26.13,44.35 23.88,46.61 R17.2
SIM_VDD  (via drill 0.61)
  Top 0.406: U2.29 29.13,40.94 28.57,40.39 24.13,40.39 | v24,39.12 24.13,39.24 24.13,40.39 | 24.13,40.39 20.19,44.32 C20.1
  Bottom 0.406: U4.1 16.97,38.61 23.62,38.61 24,38.99 v24,39.12
  Bottom 0.61: 23.96,39.08 v24,39.12
SRXD
  Top 0.406: J7.3 50.29,46.61 46.99,49.91 46.99,51.56 45.85,52.7 42.93,52.7 41.66,51.44 U3.9
STATUS
  Top 0.406: U2.49 18.95,24.99 18.16,25.78 18.16,33.66 16.26,35.56 12.45,35.56 11.18,36.83 11.18,40.77 10.41,41.53 R14.1
STXD
  Top 0.406: J7.4 49.28,45.59 49.28,46.48 45.72,50.04 U3.8
TXD
  Top 0.406: U2.14 44.18,35.94 47.75,35.94 48.9,34.8 55.24,34.8 55.88,35.43 R33.1 55.81,36.64 Q8.2 55.94,38.35 57.4,38.35 59.56,40.51 62.36,40.51 63.37,41.53 J1.8
VBAT
  Top 0.61: 47.37,27.56 46.94,27.99 U2.6 43.81,27.67 43.81,27.56 43.43,27.94 43.43,26.42 43.69,26.16 46.86,26.16 47.12,26.42 47.12,27.05 | U2.4 47.7,25.99 47.94,26.23
  Top 0.813: 56.77,9.14 56.77,9.02
  Top 1.016: R4.2 C5.2 | R5.2 C5.2 | U1.4 55.24,13.59 56.77,12.06 56.77,9.14 56.9,9.02 | C5.2 56.77,9.02 56.9,9.02 | 57.91,9.02 56.9,9.02
  Top 1.27: U1.4 48.51,13.59 C4.+ | 47.12,27.05 44.19,27.05 U2.5
  Top 1.778: VBAT.1 64.52,6.1 61.59,9.02 57.91,9.02 57.4,9.02 | C4.+ 48.45,25.72 47.94,26.23 47.12,27.05
VDD_EXT  (via drill 0.41, 0.6)
  Top 0.406: v48.64,28.96 44.16,28.96 U2.7 44.1,28.96 34.67,28.96 | R30.1 50.1,36.76 Q7.1 51.12,39.24 52.83,39.24 53.85,38.23 Q8.1 | R33.2 53.91,37.02 Q8.1 | J1.10 62.1,45.59 59.44,45.59 57.28,43.43 57.28,40.01 56.52,39.24 54.99,39.24 53.98,38.23 Q8.1 | v34.67,21.34 34.67,28.96 | 34.67,28.96 v34.67,35.05 | R8.1 v18.54,43.43
  Bottom 0.406: v48.64,28.96 61.47,28.96 63.25,30.73 63.25,32.77 65.15,34.67 65.15,42.8 63.63,44.32 J1.9 J1.10 | J2.6 23.5,21.21 34.54,21.21 v34.67,21.34 | v34.67,35.05 34.67,39.75 33.15,41.27 20.7,41.27 v18.54,43.43
VIN  (via drill 0.38 pad 0.81, 0.6)
  Top 0.406: PWR.+ D7.+ 1.14,47.88 0.64,47.37 0.64,41.66 | D2.+ 0.76,41.53 0.64,41.66 | 54.48,25.91 54.61,26.04 | 55.24,22.61 55.5,22.86 56.13,22.86 | 0.64,41.66 0.64,38.35 1.14,37.85 D3.+ | 52.58,22.99 53.09,22.99 53.09,22.48 | 53.59,22.48 v53.59,22.99 | 52.96,22.48 52.45,22.48 v52.45,22.1 | 52.96,22.23 52.96,22.35 52.96,22.48 | 52.96,22.23 52.45,22.23 v52.45,22.1 | 53.09,22.48 53.59,22.48 | 53.59,22.48 v53.59,22.1 | 53.09,22.48 52.96,22.48 | 52.96,22.23 52.96,21.84 | 52.32,22.1 v52.45,22.1 | 53.09,22.1 v52.45,22.1 | v52.45,22.1 v52.45,22.99 52.58,22.99 | 52.58,22.99 53.09,22.48 | 42.29,12.83 41.78,12.83 v41.66,12.7 | 42.67,13.72 42.67,13.84 v42.8,13.84 | v42.8,13.84 42.8,12.83 42.93,12.7 42.93,13.46 42.67,13.72 | 42.67,13.72 v42.8,13.84 | 42.04,13.46 42.67,13.72
  Top 0.61: 55.24,22.61 55.37,22.48 | C1.2 C2.2 | 54.48,25.91 R7.2 | 54.61,26.04 C2.2 | 56.13,22.86 C2.2 | D6.- 38.41,9.65 42.16,9.65 42.29,9.78 42.29,12.7 | 42.29,12.83 42.29,12.95 | v20.32,51.31 2.92,51.31 2.03,50.42 PWR.+
  Top 0.813: U1.2 51.56,16.89 51.56,18.54 U1.1 | U1.1 53.98,18.54 | 54.1,18.54 53.98,18.54 | 53.98,18.54 53.98,17.02 53.59,17.02 53.59,17.27 | 53.59,17.53 53.59,18.29 52.07,18.29 | 51.94,18.29 52.07,18.29 | 52.07,18.29 52.07,17.27 53.59,17.27 | 53.59,17.27 53.59,17.53 | 53.59,17.53 52.2,17.53 52.2,17.78 52.83,17.78 U1.1
  Top 1.778: D6.- D5.- 42.29,12.7 42.29,12.83 | U1.1 52.83,22.23 52.96,22.35 53.09,22.48 55.37,22.48 59.69,22.48 C3.+
  Bottom 0.406: v41.66,12.7 42.29,12.7 | 42.29,12.83 42.67,12.83 | 42.67,12.83 42.8,12.83 | 42.8,12.83 v42.8,12.7 | 42.29,12.83 42.29,13.21 | 42.29,12.83 41.78,12.83 v41.66,12.7 | v41.66,12.7 41.78,12.57 42.29,12.57 42.29,12.7 | 42.29,12.83 42.29,12.7 | 42.8,12.57 v42.8,12.7 | v42.8,12.7 42.67,12.83 | 42.67,12.83 42.04,13.08 | 53.09,22.48 v52.45,22.1 | 42.67,13.84 42.67,13.72 v42.8,13.84 42.67,13.84 | 42.67,13.84 v41.66,13.84 42.8,13.08 42.8,12.83 | 42.8,12.83 42.55,13.21
  Bottom 0.61: 42.29,12.95 42.29,13.21 42.29,35.05 28.96,48.39 23.24,48.39 v20.32,51.31
  Bottom 1.778: 42.29,12.83 42.29,12.95
  Bottom 1.93: 42.55,13.21 48.9,13.21 53.09,17.4 53.09,22.48
VRTC  (via drill 0.61)
  Top 0.61: U2.17 v46.23,38.99 C6.2
  Bottom 0.61: J14.+ 45.03,38.99 v46.23,38.99
(copper drawn outside any net)
  shapes: Bottom area x3, Top area x3

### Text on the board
tPlace: GPRS_RX | SWserial | GND | VDD_EXT | Xduino | 1PPS | RI | GPRS_TX | DCD | Status | TXD | CTS | RXD | RTS | DTR | NetLight | PWM1 | GPIO6 | GPIO5 | PWM2 | ADC1 | SCL | ADC2 | SDA | GND | VDD_EXT | GND | 4.2V
bPlace: 3V CR1220 | SIMHOLDER | SIM Card Holder | GPRS+GSM+GPS Shield | v1.0 2015/07/2 | www.elecrow.com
